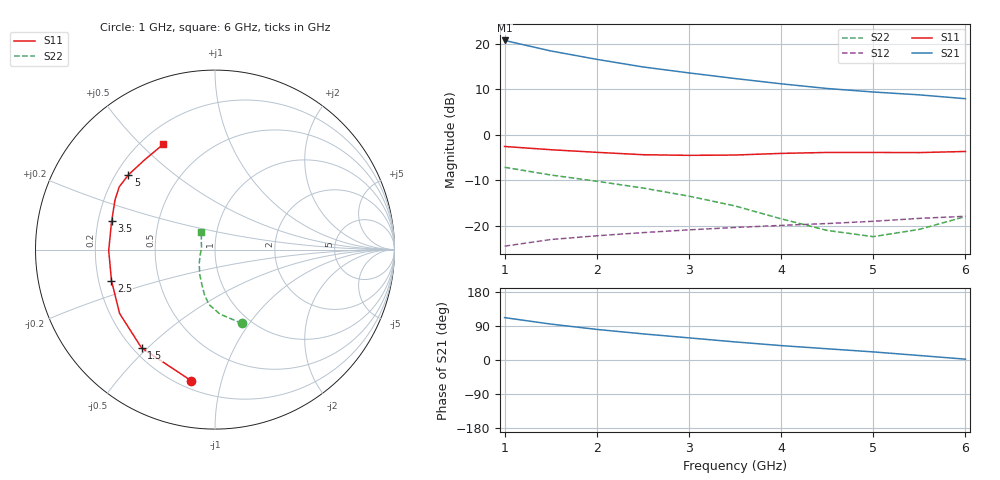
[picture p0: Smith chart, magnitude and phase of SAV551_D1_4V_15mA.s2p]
! Created Mon Oct 27 14:30:41 2008
# hz S ma R 50
! 2 Port Network Data from SP1.SP block
! freq  magS11  angS11  magS21  angS21  magS12  angS12  magS22  angS22
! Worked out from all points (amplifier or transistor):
!   11 points, 1 GHz to 6 GHz, reference 50 ohm
!   highest |S21| = 20.8 dB at 1 GHz (marker M1)
!   |S21| within 3 dB of that: start of sweep to 1.687 GHz
!   unconditionally stable (mu >= 1): 4.5 GHz to end of sweep
!   at 1.5 GHz: K = 0.46, MSG = 20.8 dB, |S12| = -23.1 dB
!   at 3.5 GHz: K = 0.90, MSG = 16.4 dB, |S12| = -20.4 dB
!   at 6 GHz: K = 1.09, MAG = 11.2 dB, |S12| = -18.0 dB
!   S11 on the Smith chart (normalised r, x): 1 GHz: 0.25, -0.80; 1.5 GHz: 0.23, -0.48; 2.5 GHz: 0.25, -0.14; 3.5 GHz: 0.26, +0.13; 5 GHz: 0.25, +0.35; 6 GHz: 0.29, +0.59
1e9  0.742 -100.3  10.91 111.8  0.05921 39.9  0.4379 -70.0
1.5e9  0.6834 -126.8  8.371 94.8  0.07007 31.0  0.36 -85.7
2e9  0.6397 -146.2  6.76 80.7  0.07705 25.0  0.3073 -96.3
2.5e9  0.6021 -163.3  5.578 69.0  0.08347 20.5  0.2588 -103.1
3e9  0.5922 -179.5  4.793 58.4  0.08954 17.5  0.2106 -110.1
3.5e9  0.5973 164.7  4.156 47.8  0.0951 13.4  0.1642 -121.1
4e9  0.6224 153.5  3.637 38.0  0.1003 9.7  0.1185 -138.1
4.5e9  0.6379 146.8  3.227 29.6  0.1051 6.3  0.08828 -159.7
5e9  0.6374 139.1  2.954 21.4  0.1113 4.2  0.07536 174.0
5.5e9  0.6356 128.1  2.747 11.9  0.1198 0.0  0.09064 147.3
6e9  0.6537 116.2  2.491 2.2  0.1264 -5.1  0.1254 126.9
